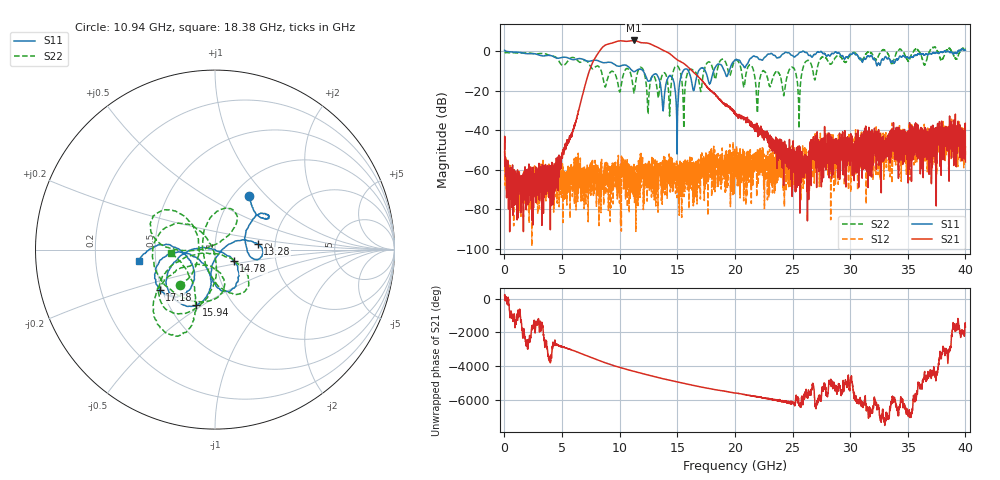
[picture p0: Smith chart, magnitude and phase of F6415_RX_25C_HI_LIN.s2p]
!Keysight Technologies,N5245B,MY52451815,A.15.70.20
!Date: Wednesday, April 17, 2024 14:35:25
!Correction: S33(C  2-Port  )
!S43(C  2-Port  )
!S34(C  2-Port  )
!S44(C  2-Port  )
!S2P File: Measurements: S33, S43, S34, S44:
# Hz S  RI  R 50
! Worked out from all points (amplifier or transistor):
!   4000 points, 10 MHz to 40 GHz, reference 50 ohm
!   highest |S21| = 5.5 dB at 11.21 GHz (marker M1)
!   |S21| within 3 dB of that: 8.594 GHz to 13.1 GHz (4.506 GHz wide, 41.5 % of centre)
!   unconditionally stable (mu >= 1): 149.6 MHz to 25.87 GHz; 25.98 GHz to 32.69 GHz; 35.96 GHz to 36.91 GHz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
!   at 6.67 GHz: K = 7089.48, MAG = -20.7 dB, |S12| = -66.2 dB
!   at 20.01 GHz: K = 3869.86, MAG = -28.4 dB, |S12| = -53.1 dB
!   at 40 GHz: K = 2810.85, MSG = -4.1 dB, |S12| = -48.0 dB
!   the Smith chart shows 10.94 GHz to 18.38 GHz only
!   S11 on the Smith chart (normalised r, x): 10.94 GHz: 1.17, +0.80; 13.28 GHz: 1.62, +0.10; 14.78 GHz: 1.22, -0.16; 15.94 GHz: 0.68, -0.47; 17.18 GHz: 0.49, -0.26; 18.38 GHz: 0.40, -0.06
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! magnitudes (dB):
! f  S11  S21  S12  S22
! 10 MHz  0.5  -49.5  -50.4  -0.7
! 1.4 GHz  -0.6  -69.3  -67.8  -0.9
! 4.05 GHz  -2.2  -66.7  -61.6  -2.3
! 6.68 GHz  -3.8  -24.3  -71.4  -5.4
! 8.41 GHz  -5.5  1.3  -68.3  -10.1
! 10.94 GHz  -9.0  5.3  -70.3  -11.1
! 11.21 GHz  -10.3  5.5  -73.7  -20.3
! 11.85 GHz  -9.3  4.4  -51.8  -8.2
! 13.28 GHz  -12.4  2.0  -58.0  -21.1
! 13.34 GHz  -13.2  1.8  -57.3  -23.4
! 14.78 GHz  -18.2  -3.4  -67.0  -8.1
! 15.56 GHz  -9.4  -6.2  -68.7  -38.9
! 15.94 GHz  -9.7  -8.1  -63.8  -10.2
! 17.18 GHz  -8.4  -15.1  -60.6  -14.6
! 18.38 GHz  -7.3  -22.4  -55.1  -12.2
! 20.01 GHz  -4.4  -32.0  -53.1  -4.9
! 21.95 GHz  -2.9  -39.0  -57.1  -31.3
! 24.94 GHz  -2.1  -55.4  -50.6  -8.1
! 25.44 GHz  -1.8  -52.5  -53.9  -16.8
! 26.67 GHz  -2.9  -48.7  -46.5  -7.6
! 33.34 GHz  -3.5  -51.1  -60.5  -2.0
! 40 GHz  0.4  -56.1  -48.0  1.2
